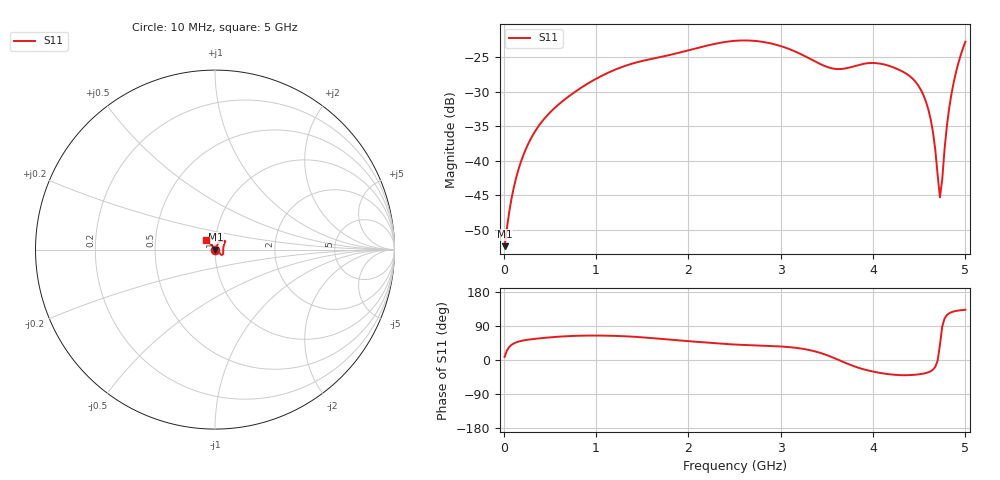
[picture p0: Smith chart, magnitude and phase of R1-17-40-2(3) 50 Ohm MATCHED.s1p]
!version-1
!date-02.2022
!Test device: УЛ34.1651.00
#	GHZ	S	RI	R	50.0
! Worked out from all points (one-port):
!   200 points, 10 MHz to 5 GHz, reference 50 ohm
!   lowest |S11| = -52.4 dB at 10 MHz (marker M1), VSWR 1.00, Z = 50.2 + j0.035 ohm
!   |S11| at or under -10 dB: start of sweep to end of sweep
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0.01  0.00238 0.000349
0.0601508  0.00352 0.00241
0.0852261  0.00408 0.00343
0.135377  0.00519 0.00548
0.210603  0.00677 0.0085
0.386131  0.00984 0.0152
0.636884  0.0126 0.0238
0.937789  0.016 0.0335
1.26377  0.0213 0.0421
1.89065  0.0373 0.0473
2.51754  0.056 0.0481
2.84352  0.0568 0.0437
3.14442  0.0523 0.0336
3.54563  0.0462 0.00694
3.77131  0.0462 -0.0119
4.07221  0.0419 -0.0282
4.39819  0.0314 -0.0262
4.52357  0.0256 -0.0192
4.59879  0.0198 -0.0126
4.64894  0.0145 -0.00693
4.67402  0.0114 -0.00371
4.72417  0.0042 0.00344
4.74925  0.000196 0.00733
4.77432  -0.00405 0.0114
4.7994  -0.00852 0.0157
4.84955  -0.018 0.0246
4.92477  -0.0332 0.0388
5  -0.0491 0.0536
